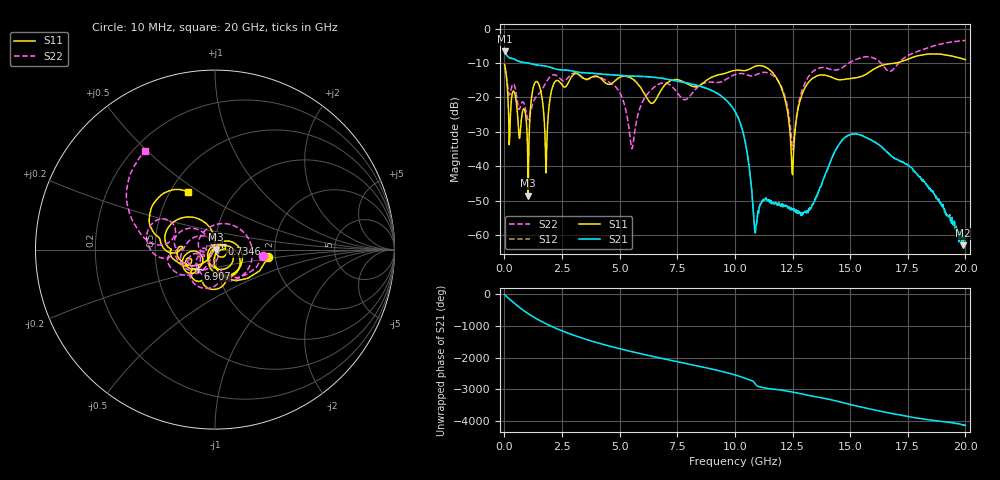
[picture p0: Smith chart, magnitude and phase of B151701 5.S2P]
!  2-Port S-parameters saved by WinCal
! VAR MeasName=S-Parameters (CALIBRATED_DATA) read from VNA (N5244A)
! VAR MeasDate=2015-12-24 19:08:44
! VAR NAME=B151701 5
! VAR FILENAME=B151701 5.S2P
! VAR DATE=2015-12-24 19:08:44
! VAR PHYS_PORTS=1,3
# Hz S DB R 50
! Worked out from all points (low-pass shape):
!   801 points, 10 MHz to 20 GHz, reference 50 ohm
!   highest |S21| = -6.62 dB at 10 MHz (marker M1); lowest = -62.9 dB at 19.9 GHz (marker M2)
!   |S21| within 3 dB of the highest: start of sweep to 667.7 MHz
!   lowest |S11| = -48.5 dB at 1.034 GHz (marker M3), VSWR 1.01, Z = 50.4 + j0.0294 ohm
!   |S11| at or under -10 dB: start of sweep to 16.98 GHz
!   |S22| runs from -35.1 to -3.5 dB; largest |S21 - S12| = 0.00099
!   S11 on the Smith chart (normalised r, x): 10 MHz: 1.83, -0.17; 734.6 MHz: 1.07, +0.06; 6.907 GHz: 0.81, -0.17; 20 GHz: 0.61, +0.45
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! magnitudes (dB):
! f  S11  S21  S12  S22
! 10 MHz  -10.5  -6.6  -6.6  -11.4
! 209.9 MHz  -33.7  -8.5  -8.4  -19.3
! 734.6 MHz  -26.6  -9.7  -9.7  -21.8
! 1.034 GHz  -48.5  -10.0  -10.0  -26.5
! 1.359 GHz  -15.4  -10.5  -10.5  -20.0
! 1.809 GHz  -41.9  -10.9  -10.9  -15.7
! 2.184 GHz  -15.6  -11.7  -11.7  -13.4
! 3.358 GHz  -14.0  -12.8  -12.8  -14.2
! 4.883 GHz  -14.7  -13.5  -13.5  -17.4
! 5.532 GHz  -14.5  -13.8  -13.8  -34.9
! 6.682 GHz  -19.3  -14.3  -14.3  -16.2
! 6.907 GHz  -16.8  -14.5  -14.5  -15.8
! 10.01 GHz  -12.1  -24.1  -24.0  -13.4
! 10.48 GHz  -12.2  -34.1  -34.0  -13.3
! 10.88 GHz  -11.0  -59.1  -59.8  -13.5
! 11.95 GHz  -16.2  -51.2  -51.2  -16.0
! 12.5 GHz  -42.5  -52.6  -52.3  -35.1
! 13.35 GHz  -14.5  -51.2  -51.1  -12.6
! 14.8 GHz  -14.7  -31.5  -31.4  -10.7
! 16.68 GHz  -10.2  -36.3  -36.3  -12.4
! 19.9 GHz  -8.8  -62.9  -61.7  -3.5
! 20 GHz  -9.0  -60.3  -62.2  -3.5
